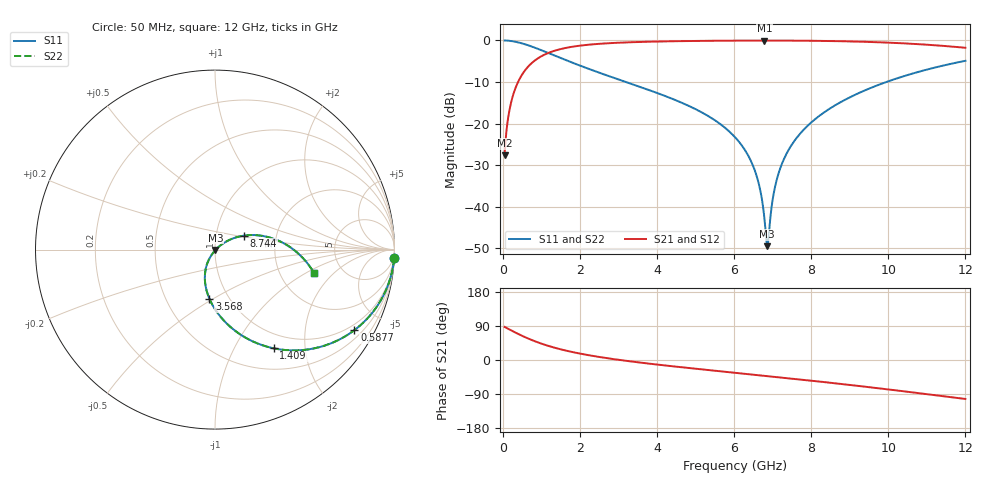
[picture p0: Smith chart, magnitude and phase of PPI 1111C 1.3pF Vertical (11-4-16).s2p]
# GHz S MA R 50
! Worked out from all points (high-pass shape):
!   1601 points, 50 MHz to 12 GHz, reference 50 ohm
!   highest |S21| = -0.03 dB at 6.787 GHz (marker M1); lowest = -27.6 dB at 50 MHz (marker M2)
!   |S21| within 3 dB of the highest: 1.178 GHz to end of sweep
!   lowest |S11| = -49.4 dB at 6.862 GHz (marker M3), VSWR 1.01, Z = 50.2 - j0.246 ohm
!   |S11| at or under -10 dB: 3.198 GHz to 9.947 GHz (6.749 GHz wide, 103 % of centre)
!   |S22| runs from -49.4 to 0.0 dB; largest |S21 - S12| = 0
!   S11 on the Smith chart (normalised r, x): 50 MHz: 1, -42; 587.8 MHz: 0.78, -3.57; 1.409 GHz: 0.78, -1.46; 3.568 GHz: 0.81, -0.48; 8.744 GHz: 1.36, +0.22; 12 GHz: 3.11, -1.22
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0.05  0.9991 -2.7  0.04178 87.3  0.04178 87.3  0.9991 -2.7
0.1545625  0.9917 -8.4  0.1282 81.6  0.1282 81.6  0.9917 -8.4
0.2516563  0.9785 -13.5  0.206 76.5  0.206 76.5  0.9785 -13.5
0.58775  0.8968 -30.1  0.4419 59.9  0.4419 59.9  0.8968 -30.1
1.409312  0.6403 -59.2  0.7669 30.7  0.7669 30.7  0.6403 -59.2
2.044156  0.4904 -73.7  0.87 16.1  0.87 16.1  0.4904 -73.7
3.567781  0.2759 -96.4  0.959 -6.8  0.959 -6.8  0.2759 -96.4
4.038312  0.2305 -101.9  0.9707 -12.4  0.9707 -12.4  0.2305 -101.9
5.255719  0.1293 -114.5  0.9887 -25.7  0.9887 -25.7  0.1293 -114.5
6.025  0.06875 -121.2  0.9943 -33.7  0.9943 -33.7  0.06875 -121.2
6.532875  0.02788 -122.3  0.9961 -38.9  0.9961 -38.9  0.02788 -122.3
6.68225  0.01567 -118.4  0.9962 -40.5  0.9962 -40.5  0.01567 -118.4
6.786812  0.007359 -104.7  0.9963 -41.6  0.9963 -41.6  0.007359 -104.7
6.8615  0.003371 -46.6  0.9963 -42.4  0.9963 -42.4  0.003371 -46.6
6.906313  0.004913 3.7  0.9962 -42.8  0.9962 -42.8  0.004913 3.7
7.048219  0.01613 33.3  0.996 -44.3  0.996 -44.3  0.01613 33.3
7.234938  0.03229 37.4  0.9955 -46.3  0.9955 -46.3  0.03229 37.4
7.556094  0.06118 36.8  0.994 -49.7  0.994 -49.7  0.06118 36.8
8.019156  0.105 33.1  0.9901 -54.7  0.9901 -54.7  0.105 33.1
8.743625  0.179 25.8  0.979 -62.8  0.979 -62.8  0.179 25.8
10.01331  0.3242 11.3  0.9403 -77.8  0.9403 -77.8  0.3242 11.3
12  0.5688 -13.5  0.8155 -102.8  0.8155 -102.8  0.5688 -13.5
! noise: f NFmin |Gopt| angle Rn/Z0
0.05  0.0008314  0.9604  2.105  0.004738
1.372  0.004319  0.7164  11.72  0.002978
2.701  0.006879  0.6612  19.47  0.003777
4.031  0.00921  0.6356  27.14  0.004511
5.36  0.01149  0.6258  34.51  0.00527
6.682  0.01382  0.6268  41.46  0.006115
8.012  0.01632  0.6362  48.03  0.00712
9.341  0.01906  0.6524  54.21  0.00836
10.67  0.02215  0.6739  60.03  0.009941
12  0.02574  0.6998  65.53  0.01202
